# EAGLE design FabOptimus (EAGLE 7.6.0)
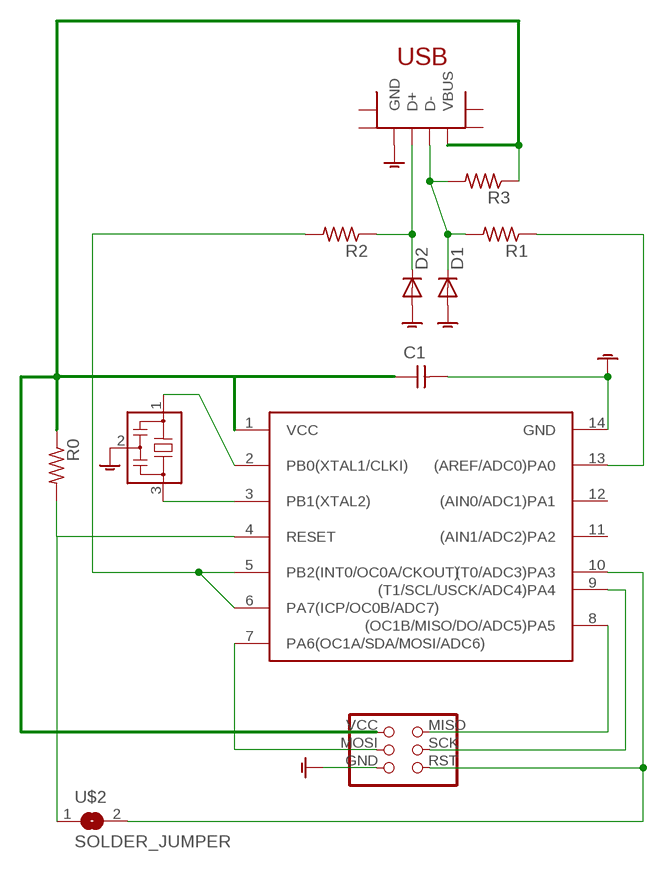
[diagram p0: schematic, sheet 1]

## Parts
C1  CAP-UNPOLARIZEDFAB  [C1206FAB]
D1  DIODESOD123  [SOD123]
D2  DIODESOD123  [SOD123]
IC1  ATTINY44-SSU  [SOIC14_ATTTINY44]
JP1  2X3PINHEADER  [2X3PINHEADER]
R0  RES-US1206FAB  [R1206FAB]
R1  RES-US1206FAB  [R1206FAB]
R2  RES-US1206FAB  [R1206FAB]
R3  RES-US1206FAB  [R1206FAB]
U$1  RESONATOR  [EFOBM]
U$2  SOLDER_JUMPER  [SOLDERJUMPER]
U$8  USB_MINIB  [USB_MINIB]

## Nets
GND: C1.2 D1.ANODE(A) D2.ANODE(A) IC1.14(GND) JP1.GND U$1.2 U$8.GND
N$1: IC1.2(PB0(XTAL1/CLKI)) U$1.1
N$2: D2.CATHODE(C) R2.1 U$8.D+
N$3: IC1.9((T1/SCL/USCK/ADC4)PA4) JP1.SCK
N$4: D1.CATHODE(C) R1.2 R3.2 U$8.D-
N$5: IC1.7(PA6(OC1A/SDA/MOSI/ADC6)) JP1.MOSI
N$6: IC1.5(PB2(INT0/OC0A/CKOUT)) IC1.6(PA7(ICP/OC0B/ADC7)) R2.2
N$7: IC1.3(PB1(XTAL2)) U$1.3
N$8: IC1.13((AREF/ADC0)PA0) R1.1
N$9: IC1.8((OC1B/MISO/DO/ADC5)PA5) JP1.MISO
N$10: IC1.10((T0/ADC3)PA3) JP1.RST U$2.2
N$11: IC1.4(RESET) R0.2 U$2.1
R4: C1.1 IC1.1(VCC) JP1.VCC R0.1 R3.1 U$8.V(VBUS)
Unconnected: IC1.11((AIN1/ADC2)PA2) IC1.12((AIN0/ADC1)PA1) U$8.SHIELD@1(SHIELD) U$8.SHIELD@2(SHIELD1) U$8.SHIELD@3(SHIELD2) U$8.SHIELD@4(SHIELD3)

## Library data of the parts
C1 = fab:CAP-UNPOLARIZED
D1 D2 = fab:DIODE: DIODE
IC1 = myFab:ATTINY44
JP1 = myFab:2X3PINHEADER: PIN HEADER
R0 R1-R3 = fab:RES-US: Resistor (US Symbol)
U$1 = fab:RESONATOR
U$2 = myFab:SOLDER_JUMPER
U$8 = myFab:USB_MINIB

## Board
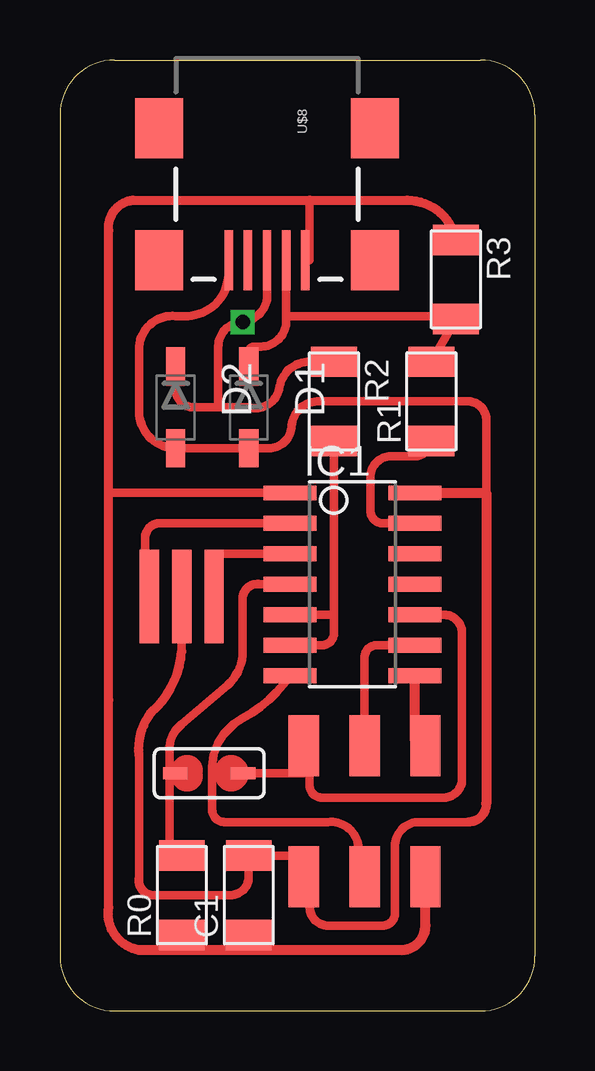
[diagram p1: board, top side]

Size 19.81 x 39.62 mm. Coordinates in mm from the lower left corner, seen from the top.
Outline: 2.29,39.62 17.53,39.62 arc-90 19.81,37.34 19.81,2.29 arc-90 17.53,0 2.29,0 arc-90 0,2.29 0,37.34 arc-90 2.29,39.62
Copper layers (1*16): Top 0.035mm / dielectric 1.5mm / Bottom 0.035mm
Design rules "default": minimum track width 10mil, minimum drill 24mil, track to track 8mil, track to pad 8mil, pad to pad 8mil, via to via 8mil, smd to smd 8mil, copper to edge 40mil, drill to drill 8mil, minimum pad ring 10mil, minimum via ring 8mil, stop-mask expansion 4mil, vias tented up to drill 0mil, thermal gap 10mil

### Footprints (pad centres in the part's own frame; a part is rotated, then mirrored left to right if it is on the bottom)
C1206FAB = smd 1.27 x 1.905: 1 -1.651,0; 2 1.651,0
SOD123 = smd 1.6 x 0.8: ANODE 1.7,0; CATHODE -1.7,0
SOIC14_ATTTINY44 = smd 2.21 x 0.61: 1 -3.873,3.81; 2 -3.873,2.54; 3 -3.873,1.27; 4 -3.873,0; 5 -3.873,-1.27; 6 -3.873,-2.54; 7 -3.873,-3.81; 8 1.333,-3.81; 9 1.333,-2.54; 10 1.333,-1.27; 11 1.333,0; 12 1.333,1.27; 13 1.333,2.54; 14 1.333,3.81
2X3PINHEADER = smd 2.54 x 1.27: GND -2.54,2.54; MISO 2.92,-2.54; MOSI -2.54,0; RST 2.92,2.54; SCK 2.92,0; VCC -2.54,-2.54
R1206FAB = smd 1.27 x 1.905: 1 -1.651,0; 2 1.651,0
EFOBM = smd 0.8 x 3.9: 1 -1.35,0; 2 0,0; 3 1.35,0
SOLDERJUMPER = smd 1.016 x 0.508: 1 -2.057,0; 2 0.787,0
USB_MINIB = smd 2.5 x 0.35: D+ 3.77,0; D- 3.77,0.8; GND 3.77,-1.6; ID 3.77,-0.8; V 3.77,1.6 | smd 2.5 x 2: SHIELD@1 -1.73,-4.5; SHIELD@2 -1.73,4.5; SHIELD@3 3.77,4.5; SHIELD@4 3.77,-4.5

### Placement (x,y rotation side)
C1  7.87,4.83 90 top
D1  7.87,25.15 270 top
D2  4.83,25.15 270 top
IC1  13.46,17.78 0 top
JP1  12.7,8.13 90 top
R0  5.08,4.83 90 top
R1  15.49,25.4 90 top
R2  11.43,25.4 270 top
R3  16.51,30.48 270 top
U$1  5.08,17.27 0 top
U$2  6.86,9.91 0 top
U$8  8.64,35.05 270 top

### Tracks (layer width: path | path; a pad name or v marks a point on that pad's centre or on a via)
GND
  Top 0.356: 15.49,21.59 IC1.14 | 17.02,7.87 14.99,7.87 arc90 13.97,6.86 13.97,4.06 arc-90 13.46,3.56 11.18,3.56 arc-90 10.41,4.32 10.41,4.57 arc90 10.16,4.83 arc90 9.91,4.83 | 3.3,10.67 3.3,5.59 arc90 3.81,4.83 7.11,4.83 arc90 7.87,5.59 C1.2 10.16,6.48 JP1.GND | 17.78,21.59 17.78,24.64 arc90 17.02,25.4 10.92,25.4 arc90 9.65,24.38 arc-90 8.71,23.45 D1.ANODE D2.ANODE arc-90 3.3,24.97 3.3,27.69 arc-90 4.83,28.96 5.33,28.96 arc62 6.86,29.97 arc29 U$8.GND | 5.08,14.99 U$1.2
  Top 0.381: 17.78,8.64 arc-90 17.02,7.87 | 3.3,10.67 arc-44 3.81,12.45 arc44 5.08,14.99
  Top 0.406: 10.16,4.83 JP1.GND | 17.78,8.64 17.78,21.59 15.49,21.59
N$1
  Top 0.356: IC1.2 4.06,20.32 arc90 3.56,19.56 3.56,17.1 arc-90 U$1.1
N$2  (via drill 0.6)
  Top 0.356: R2.1 10.54,27.05 arc90 9.14,25.91 arc-90 7.87,25.15 6.6,25.15 | D2.CATHODE 4.83,25.91 arc90 5.59,25.15 6.6,25.15 | U$8.D+ 8.64,29.97 arc-90 v7.62,28.7 arc90 6.6,27.69 6.6,25.15
N$3
  Top 0.356: JP1.SCK 12.7,14.73 arc-90 13.21,15.24 IC1.9
N$4
  Top 0.356: D1.CATHODE 7.87,27.43 arc-90 8.13,27.69 8.38,27.69 arc90 9.44,28.74 9.44,28.96 | 9.44,28.96 U$8.D- | 9.44,28.96 15.49,28.96 R3.2 R1.2
N$5
  Top 0.356: 9.14,13.97 IC1.7 arc-28 7.62,12.19 arc34 6.6,11.18 arc28 6.35,10.16 6.35,8.38 arc90 6.86,7.87 11.18,7.87 arc-90 12.45,6.86 JP1.MOSI
N$6
  Top 0.356: IC1.5 11.43,16.51 | 11.43,16.51 11.43,16 11.43,15.75 arc-90 10.92,15.24 IC1.6 | R2.2 11.43,16.51
N$7
  Top 0.356: IC1.3 6.35,19.05 6.35,17.35 arc90 U$1.3
N$8
  Top 0.356: IC1.13 13.46,20.32 arc-90 12.95,20.83 12.95,22.1 arc-90 13.72,23.11 14.61,23.11 arc90 R1.1
N$9
  Top 0.406: JP1.MISO 14.8,11.3 IC1.8
N$10
  Top 0.356: IC1.10 16,16.51 arc-90 16.76,15.75 16.76,9.65 arc-90 16,8.89 10.92,8.89 arc-90 10.41,9.4 10.41,10.79 arc90 JP1.RST 10.16,9.91 U$2.2
  Top 0.406: JP1.RST 10.44,11.05
N$11
  Top 0.356: IC1.4 8.38,17.78 arc90 7.62,17.27 7.62,14.99 arc-53 6.86,13.46 5.08,11.94 arc53 4.57,10.92 4.57,10.14 | 4.57,10.14 4.57,6.98 arc90 R0.2 | 4.57,10.14 arc90 U$2.1
R4
  Top 0.356: R0.1 5.33,2.54 | IC1.1 2.03,21.59 | C1.1 7.87,2.54 | U$8.V 10.41,31.28 10.41,33.78
  Top 0.368: 2.03,12.95 2.03,21.59 2.03,32.51 arc-90 3.05,33.78
  Top 0.381: 3.05,33.78 10.41,33.78 14.48,33.78 arc-78 R3.1 | 3.3,2.54 arc-90 2.03,4.32 2.03,12.95
  Top 0.406: JP1.VCC 15.24,3.56 arc-90 14.22,2.54 7.87,2.54 5.33,2.54 3.3,2.54

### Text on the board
Labels: USB | R_pullup | C | C | D / 3.3V | D / 3.3V | 100Ω | 100Ω | A | A | 20 / MHz | ATTiny44 | 0Ω | ISP | 10K | 1μF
